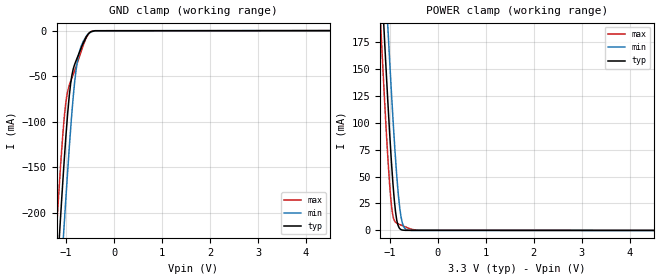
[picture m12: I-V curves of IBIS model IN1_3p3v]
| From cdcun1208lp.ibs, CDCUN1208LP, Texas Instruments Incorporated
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[Model]   IN1_3p3v
Model_type   Input
Vinl = 1.1
Vinh = 2.1
|   typ   min   max
C_comp   9.4274pF   8.4917pF   10.6224pF
[Voltage Range]   3.3   2.97   3.63
[Temperature Range]   27   105   -40
[Power Clamp Reference]   3.3   2.97   3.63
[GND Clamp Reference]   0   -0   0
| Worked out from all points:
|   GND clamp passes 1 mA (typ) near -0.46 V on its own axis
|   POWER clamp passes 1 mA (typ) near -0.77 V on its own axis
[GND Clamp]
|   Voltage   I(typ)   I(min)   I(max)
-3.3V     -2.288A    -2.351A    -2.24A
-1.212V   -287.5mA   -358.1mA   -229.8mA
-1.194V   -271.9mA   -342.6mA   -213.9mA
-1.141V   -226.1mA   -296.6mA   -168.7mA
-1.046V   -147.8mA   -218.3mA   -100.1mA
-986mV    -103.4mA   -168.9mA   -71.89mA
-906.3mV  -58.47mA   -108.3mA   -55.78mA
-856.8mV  -43.32mA   -75.49mA   -48.82mA
-794.6mV  -33.35mA   -44.06mA   -40.03mA
-685.4mV  -19.01mA   -17.09mA   -22.68mA
-466.8mV  -1.024mA   -1.26mA    -753.6uA
6.59V     0A         0A         0A
[POWER Clamp]
|   Voltage   I(typ)   I(min)   I(max)
-3.3V     2.294A     2.358A     2.243A
-1.194V   249.8mA    321.6mA    192.8mA
-1.184V   240.7mA    312.5mA    183.9mA
-1.13V    192.8mA    264.1mA    136.9mA
-1.038V   115.8mA    184.8mA    64.06mA
-964.3mV  61.45mA    125.4mA    22.2mA
-880.3mV  16.63mA    65.38mA    7.649mA
-824.3mV  4.211mA    33.44mA    6.02mA
-764.6mV  718.7uA    11.99mA    4.938mA
-685.4mV  164.3uA    1.807mA    3.503mA
-553.3mV  120.5uA    51.61uA    1.24mA
6.59V     0A         0A         0A
